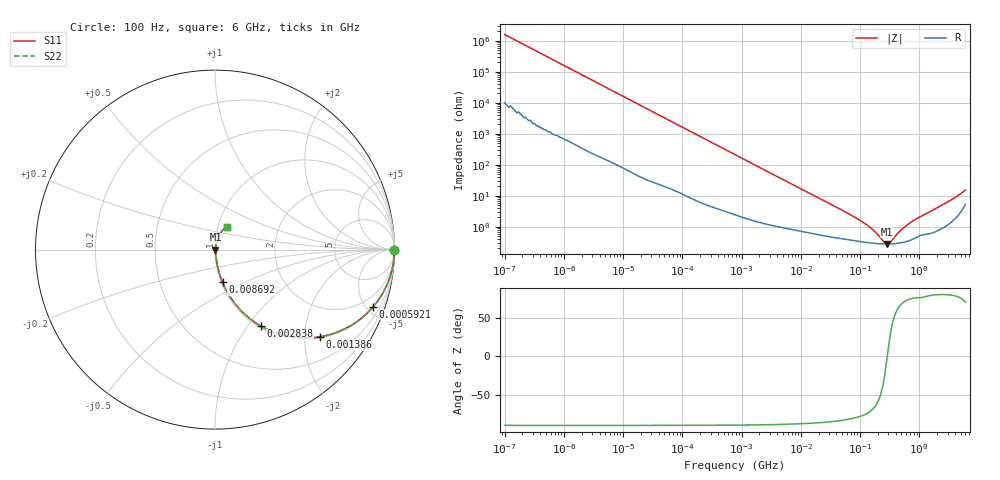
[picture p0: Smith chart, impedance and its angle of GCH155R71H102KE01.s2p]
!Murata Part Number: GCH155R71H102KE01
!These Parameters are Measured in Series Mode Connection
!Data Generated on Mar 13, 2026
!  o--ll--o
!Port1  Port2
!  o------o
!Operation Temp=25[degC], DC Bias Voltage=0[V]
!Freq. Start=100[Hz] Stop=6[GHz] 401[Steps]
# Hz S RI R 50
!Freq.(Hz) S11(Real) S11(Imag) S21(Real) S21(Imag) S12(Real) S12(Imag) S22(Real) S22(Imag)
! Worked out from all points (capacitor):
!   401 points, 100 Hz to 6 GHz, reference 50 ohm
!   read as one part in series: C = 1 nF near 109 Hz
!   lowest |Z| = 279 mohm at 285.7 MHz (marker M1)
!   series resonance near 288.1 MHz, so ESL is about 310 pH
!   S11 on the Smith chart (normalised r, x): 100 Hz: open; 592.1 kHz: 1.06, -5.52; 1.386 MHz: 1.03, -2.37; 2.838 MHz: 1.02, -1.16; 8.692 MHz: 1.02, -0.38; 6 GHz: 1.10, +0.29
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100  1 -6.29e-05  4e-07 6.29e-05  4e-07 6.29e-05  1 -6.29e-05
171  1 -0.000107  6e-07 0.000107  6e-07 0.000107  1 -0.000107
2008  1 -0.00125  6.9e-06 0.00125  6.9e-06 0.00125  1 -0.00125
40335  0.9992 -0.0249  0.000767 0.0249  0.000767 0.0249  0.9992 -0.0249
184852  0.9864 -0.112  0.0136 0.112  0.0136 0.112  0.9864 -0.112
592111  0.8815 -0.318  0.1185 0.318  0.1185 0.318  0.8815 -0.318
774597  0.8143 -0.3831  0.1857 0.3831  0.1857 0.3831  0.8143 -0.3831
1386327  0.583 -0.486  0.417 0.486  0.417 0.486  0.583 -0.486
1983483  0.4095 -0.4835  0.5905 0.4835  0.5905 0.4835  0.4095 -0.4835
2837864  0.2572 -0.4271  0.7428 0.4271  0.7428 0.4271  0.2572 -0.4271
4643984  0.1195 -0.3113  0.8805 0.3113  0.8805 0.3113  0.1195 -0.3113
8692127  0.0424 -0.1826  0.9576 0.1826  0.9576 0.1826  0.0424 -0.1826
1.555665e7  0.0174 -0.1058  0.9826 0.1058  0.9826 0.1058  0.0174 -0.1058
1.066761e8  0.00347 -0.0144  0.9965 0.0144  0.9965 0.0144  0.00347 -0.0144
1.596157e8  0.00301 -0.00785  0.997 0.00785  0.997 0.00785  0.00301 -0.00785
2.497637e8  0.00279 -0.00181  0.9972 0.00181  0.9972 0.00181  0.00279 -0.00181
2.856706e8  0.00278 -0.000105  0.9972 0.000105  0.9972 0.000105  0.00278 -0.000105
3.124326e8  0.00279 0.00103  0.9972 -0.00103  0.9972 -0.00103  0.00279 0.00103
4.888888e8  0.00307 0.00706  0.9969 -0.00706  0.9969 -0.00706  0.00307 0.00706
7.31507e8  0.00393 0.0136  0.9961 -0.0136  0.9961 -0.0136  0.00393 0.0136
3.205649e9  0.0165 0.0647  0.9835 -0.0647  0.9835 -0.0647  0.0165 0.0647
6e9  0.0672 0.1274  0.9328 -0.1274  0.9328 -0.1274  0.0672 0.1274
